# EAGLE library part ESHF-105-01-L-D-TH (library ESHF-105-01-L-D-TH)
.050" Shrouded Terminal Strip For FFSD, through hole, dual row, positions per row Source: Datasheet
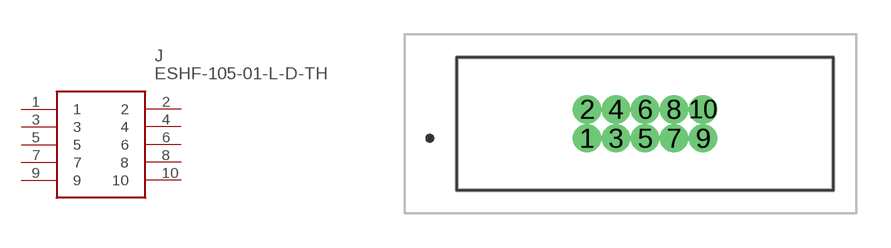
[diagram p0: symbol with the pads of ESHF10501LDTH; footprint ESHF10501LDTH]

Designator prefix J

## ESHF-105-01-L-D-TH (Arrow_Part_Number: ESHF-105-01-L-D-TH; Arrow_Price-Stock: https://www.arrow.com/en/products/eshf-105-01-l-d-th/samtec?region=nac; Description: .050" Shrouded Terminal Strip For FFSD, through hole, dual row, positions per row; Height: 5.33mm; Manufacturer_Name: SAMTEC; Manufacturer_Part_Number: ESHF-105-01-L-D-TH; Mouser_Part_Number: 200-ESHF10501LDTH; Mouser_Price-Stock: https://www.mouser.co.uk/ProductDetail/Samtec/ESHF-105-01-L-D-TH?qs=%252BZP6%2F%252BtExtA76X6DwKXxNw%3D%3D)  [ESHF10501LDTH]
1  1
2  2
3  3
4  4
5  5
6  6
7  7
8  8
9  9
10  10

## Footprint ESHF10501LDTH (pad centres in mm)
ESHF-105-01-L-D-TH-4
drill 0.74 pad 1.1: 1 0,0; 2 0,1.27; 3 1.27,0; 4 1.27,1.27; 5 2.54,0; 6 2.54,1.27; 7 3.81,0; 8 3.81,1.27; 9 5.08,0; 10 5.08,1.27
